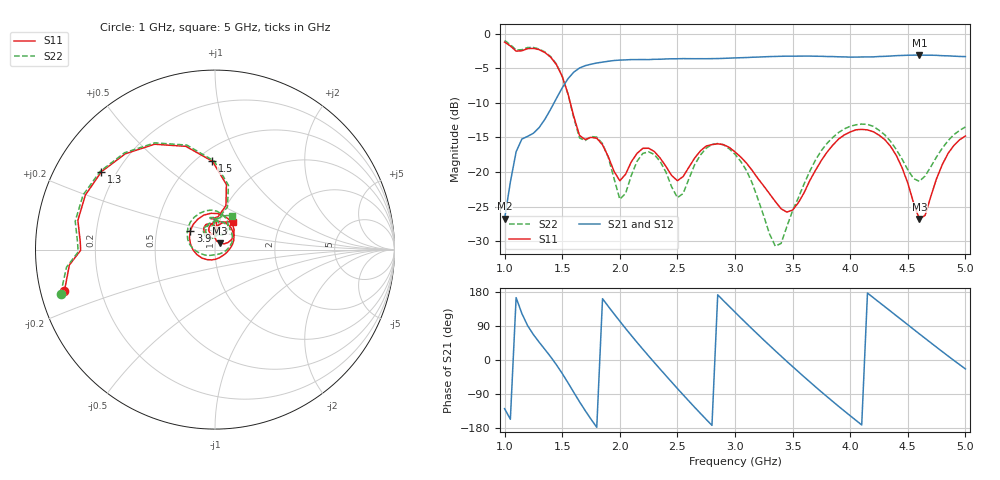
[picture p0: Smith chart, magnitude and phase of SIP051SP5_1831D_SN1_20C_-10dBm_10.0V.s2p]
# GHz  S  dB  R  50
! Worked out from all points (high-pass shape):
!   81 points, 1 GHz to 5 GHz, reference 50 ohm
!   highest |S21| = -3.09 dB at 4.6 GHz (marker M1); lowest = -26.7 dB at 1 GHz (marker M2)
!   |S21| within 3 dB of the highest: 1.572 GHz to end of sweep
!   lowest |S11| = -26.8 dB at 4.6 GHz (marker M3), VSWR 1.10, Z = 52.8 + j3.81 ohm
!   |S11| at or under -10 dB: 1.57 GHz to end of sweep
!   |S22| runs from -30.7 to -1.0 dB; largest |S21 - S12| = 0.0025
!   S11 on the Smith chart (normalised r, x): 1 GHz: 0.07, -0.13; 1.3 GHz: 0.14, +0.30; 1.5 GHz: 0.60, +0.77; 3.9 GHz: 0.74, +0.16; 5 GHz: 1.16, +0.37
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1  -1.21 -164.7  -26.73 -128.4  -26.77 -128.7  -0.97 -164.1
1.1  -2.52 -179.7  -17.06 164.6  -17.06 164.4  -2.36 -179.0
1.3  -2.30 145.6  -13.56 46.9  -13.57 47.1  -2.22 145.8
1.5  -6.16 91.6  -7.83 -35.5  -7.82 -35.4  -6.14 90.5
1.6  -11.93 76.0  -5.56 -85.3  -5.56 -85.3  -12.14 73.7
1.7  -15.30 96.0  -4.62 -133.8  -4.61 -134.0  -15.44 97.5
1.85  -16.06 88.2  -4.11 161.7  -4.10 161.7  -15.90 84.1
2.05  -20.32 118.5  -3.79 83.3  -3.79 83.4  -23.10 119.7
2.2  -16.57 110.0  -3.74 28.4  -3.74 28.4  -17.30 115.3
2.35  -17.97 88.3  -3.69 -24.0  -3.68 -24.1  -18.47 88.7
2.6  -19.29 108.4  -3.61 -108.4  -3.61 -108.5  -20.97 118.6
2.8  -16.03 82.0  -3.60 -172.5  -3.60 -172.5  -16.01 92.4
3  -17.09 44.1  -3.50 126.3  -3.49 126.2  -17.42 47.1
3.2  -20.95 8.8  -3.38 67.2  -3.37 67.1  -23.93 -2.9
3.4  -25.30 -39.5  -3.26 10.3  -3.26 10.2  -30.31 -105.4
3.7  -19.70 -163.8  -3.26 -71.2  -3.26 -71.1  -18.22 177.6
3.9  -15.22 142.6  -3.34 -122.4  -3.34 -122.4  -14.27 141.3
4.1  -13.83 96.7  -3.36 -171.4  -3.36 -171.4  -13.06 103.8
4.35  -16.28 46.2  -3.23 128.9  -3.23 128.9  -15.55 64.5
4.6  -26.80 52.0  -3.09 69.1  -3.08 69.2  -21.34 75.6
4.8  -18.90 89.2  -3.18 22.0  -3.18 22.0  -16.53 91.6
5  -14.79 56.6  -3.31 -23.6  -3.32 -23.6  -13.48 63.4
